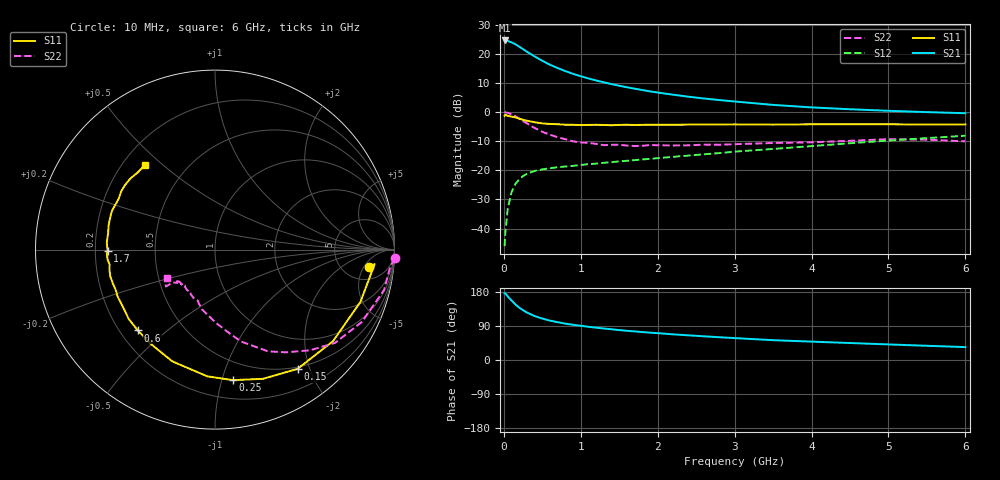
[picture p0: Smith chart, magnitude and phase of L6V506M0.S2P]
!  INFINEON TECHNOLOGIES Small Signal Semiconductors
! BFR380L3 , Si-NPN RF-Transistor in TSLP-3-1
!  Vce=0.5 V,  Ic=6 mA
! Common Emitter S-Parameters:  07. March 2005
#  GHz  S  MA  R  50
! f  S11  S21  S12  S22
! GHz  Mag  Ang  Mag  Ang  Mag  Ang  Mag  Ang
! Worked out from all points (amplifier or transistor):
!   36 points, 10 MHz to 6 GHz, reference 50 ohm
!   highest |S21| = 24.5 dB at 10 MHz (marker M1)
!   |S21| within 3 dB of that: start of sweep to 250.6 MHz
!   unconditionally stable (mu >= 1): 2.095 GHz to 5.688 GHz
!   at 250 MHz: K = 0.21, MSG = 21.8 dB, |S12| = -22.0 dB
!   at 1.4 GHz: K = 0.84, MSG = 13.4 dB, |S12| = -17.2 dB
!   at 6 GHz: K = 0.99, MSG = 3.9 dB, |S12| = -8.1 dB
!   S11 on the Smith chart (normalised r, x): 10 MHz: 9, -6; 150 MHz: 0.47, -1.81; 250 MHz: 0.34, -1.09; 600 MHz: 0.27, -0.40; 1.7 GHz: 0.25, -0.00; 6 GHz: 0.29, +0.44
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0.01  0.861 -6.4  16.85 175.9  0.005 84.4  1.003 -2.8
0.02  0.8932 -5.2  16.82 175.5  0.0087 90.6  0.9813 -5.6
0.05  0.861 -19.8  16.53 167.9  0.0217 79.8  0.9681 -13.5
0.1  0.8322 -37.8  15.62 156.9  0.0423 70.5  0.9122 -26.2
0.15  0.8081 -55.3  14.5 146.7  0.0582 62.3  0.8473 -37.8
0.2  0.7681 -69.6  13.18 138.1  0.0701 56.7  0.772 -46.6
0.25  0.7342 -82.1  11.94 131.3  0.0798 51.2  0.6953 -55.4
0.3  0.7077 -93.4  10.78 125.2  0.0871 47.8  0.6391 -62.5
0.4  0.6667 -110.9  8.948 115.9  0.0975 42.4  0.5315 -74.3
0.5  0.6368 -123.3  7.544 109.3  0.1037 39.7  0.4574 -82.1
0.6  0.6229 -133.7  6.451 103.8  0.1085 37.9  0.4073 -89.4
0.8  0.6046 -148.0  5.024 96.0  0.1161 37.6  0.3412 -102.1
0.9  0.6027 -154.0  4.5 92.9  0.1191 37.8  0.3139 -106.6
1.1  0.5996 -161.8  3.756 87.6  0.1273 39.1  0.2957 -113.6
1.4  0.5926 -171.8  3.002 81.2  0.1378 41.2  0.2735 -121.6
1.7  0.5984 -179.4  2.506 75.5  0.1494 43.9  0.261 -129.9
2.2  0.6028 170.9  1.978 67.7  0.1703 47.4  0.2667 -134.0
2.8  0.6121 161.4  1.602 60.1  0.1973 51.2  0.2742 -140.3
3.5  0.6069 152.1  1.322 52.3  0.2324 52.7  0.2939 -141.3
4.5  0.6168 144.6  1.114 44.8  0.2909 54.9  0.3205 -142.6
5.5  0.6082 135.1  0.995 37.5  0.3568 53.4  0.335 -145.1
6  0.6129 129.4  0.952 34.0  0.3913 52.1  0.3135 -149.1
